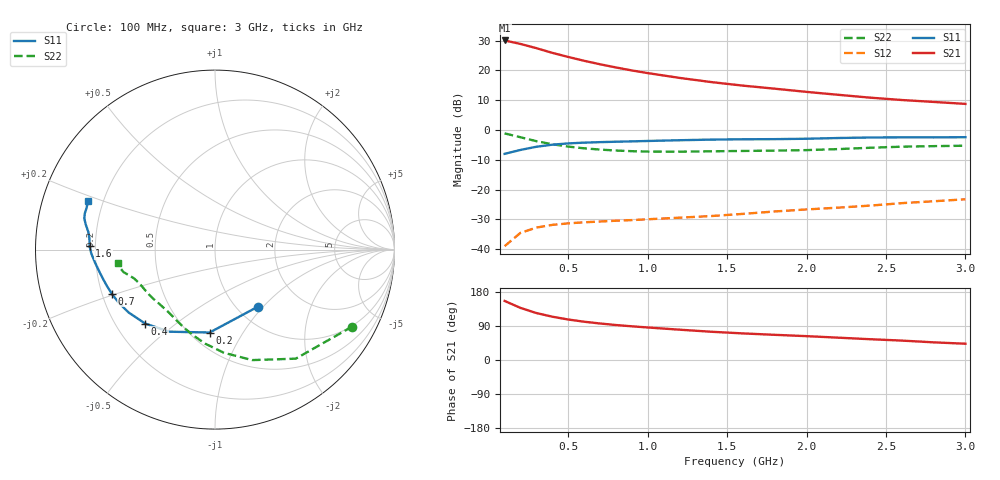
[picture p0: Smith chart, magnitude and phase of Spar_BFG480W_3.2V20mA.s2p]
! Filename: 3_220BFG480.001
! Title: BFG480W
! Bias: Vce=3.2V; Ic=20mA
! Company: NXP Semiconductors NL
! User: Quality&Reliability T&D
! Measure time: 10 Nov 1999 / 11:56:24
#  MHz  S  MA  R 50
! Freq  S11  S21  S12  S22  :
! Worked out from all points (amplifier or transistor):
!   20 points, 100 MHz to 3 GHz, reference 50 ohm
!   highest |S21| = 30.1 dB at 100 MHz (marker M1)
!   |S21| within 3 dB of that: start of sweep to 326.3 MHz
!   unconditionally stable (mu >= 1): 1.372 GHz to end of sweep
!   at 400 MHz: K = 0.39, MSG = 28.9 dB, |S12| = -31.8 dB
!   at 1.2 GHz: K = 0.94, MSG = 23.5 dB, |S12| = -29.4 dB
!   at 3 GHz: K = 1.11, MAG = 14.0 dB, |S12| = -23.3 dB
!   S11 on the Smith chart (normalised r, x): 100 MHz: 1.24, -0.94; 200 MHz: 0.62, -0.73; 400 MHz: 0.32, -0.39; 700 MHz: 0.24, -0.19; 1.6 GHz: 0.18, +0.01; 3 GHz: 0.14, +0.18
100  0.3979 -53.0  31.83 155.9  0.01123 67.4  0.8768 -29.3
200  0.4628 -93.7  27.83 137.4  0.01878 54.6  0.756 -53.5
300  0.5236 -119.1  23.63 123.9  0.02304 46.9  0.6494 -71.5
400  0.5668 -133.4  19.72 114.3  0.02556 42.5  0.5766 -85.1
500  0.5954 -144.0  16.83 106.9  0.02712 40.3  0.527 -95.9
600  0.6131 -151.3  14.51 101.0  0.02823 39.6  0.4929 -104.3
700  0.6256 -156.9  12.69 96.3  0.0291 39.9  0.4694 -111.2
800  0.6353 -161.4  11.22 92.3  0.03002 40.9  0.4524 -117.0
900  0.6444 -165.2  9.997 88.9  0.03073 42.5  0.4411 -122.1
1000  0.6542 -168.6  9.027 85.8  0.03174 44.0  0.4344 -126.7
1200  0.6735 -174.1  7.493 80.0  0.03376 47.5  0.4327 -134.7
1400  0.6895 -178.2  6.373 74.5  0.03596 51.0  0.4389 -140.9
1600  0.6992 178.4  5.555 70.2  0.03909 54.8  0.445 -145.7
1800  0.7024 175.0  4.935 66.4  0.04292 58.3  0.451 -150.4
2000  0.7131 172.0  4.364 62.9  0.04643 61.5  0.4596 -155.4
2200  0.7337 169.0  3.895 58.9  0.04974 63.5  0.4781 -160.3
2400  0.7485 166.6  3.491 54.8  0.05386 64.9  0.5035 -163.8
2600  0.7528 164.5  3.186 51.2  0.05921 66.0  0.5249 -166.2
2800  0.7522 161.9  2.958 46.6  0.06367 66.0  0.536 -168.6
3000  0.7579 159.0  2.743 42.9  0.06871 66.5  0.5447 -172.0
